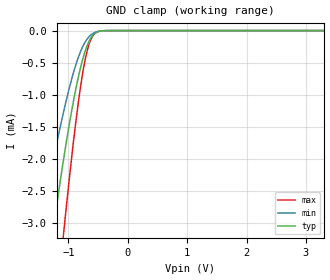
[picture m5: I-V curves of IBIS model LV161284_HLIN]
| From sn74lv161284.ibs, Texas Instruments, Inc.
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[Model]   LV161284_HLIN
Model_type  Input
Vinl=1.6
Vinh=2.6
| variable   typ   min   max
C_comp   1.13pF   0.92pF   1.33pF
[Temperature Range]   40   100   -40
| Ambient temperature   25   85   -40
[Voltage range]   3.3   3   3.6
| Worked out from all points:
|   GND clamp passes 1 mA (typ) near -0.89 V on its own axis
[GND Clamp]
| LV161284_HLIN
|   Voltage   I(typ)   I(min)   I(max)
-3.3V     -21.29mA   -14.5mA    -28.11mA
-1.505V   -4.888mA   -3.244mA   -7.411mA
-1.465V   -4.59mA    -3.039mA   -6.988mA
-1.265V   -3.175mA   -2.069mA   -4.935mA
-1.085V   -2.032mA   -1.284mA   -3.204mA
-1.055V   -1.856mA   -1.164mA   -2.93mA
-925mV    -1.152mA   -690.7uA   -1.815mA
-780mV    -521.8uA   -293.4uA   -781.8uA
-680mV    -225.2uA   -126.9uA   -301.3uA
-565mV    -51.65uA   -34.3uA    -54.54uA
-365mV    -1.323uA   -1.023uA   -624.3nA
3.3V      4.502nA    731.1pA    21.74nA
